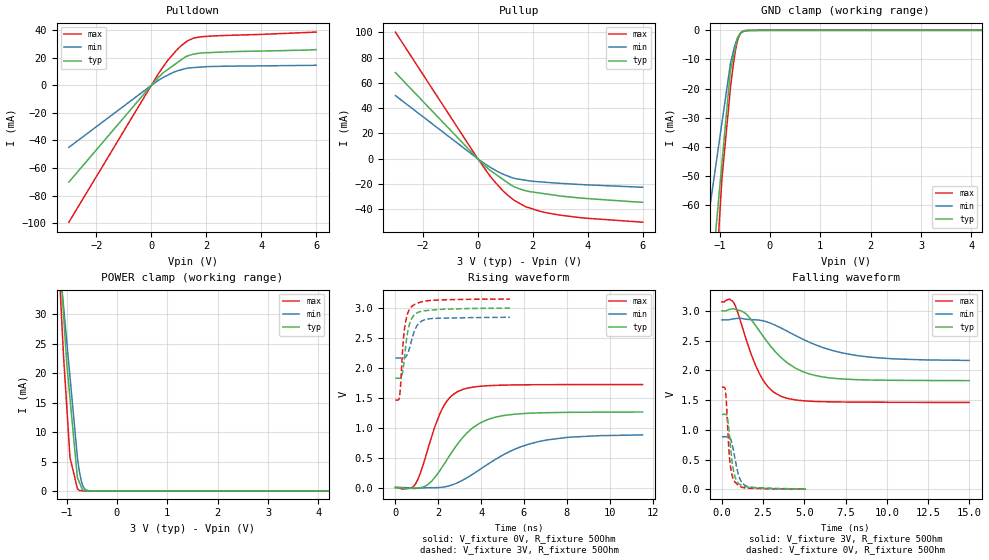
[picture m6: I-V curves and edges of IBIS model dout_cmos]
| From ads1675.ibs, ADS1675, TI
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|   dout_cmos Model
[Model]   dout_cmos
Model_type   3-state
Polarity   Non-Inverting
Vmeas = 1.5
Vref = 0
Cref = 5pF
Rref = 500
|   typ   min   max
|C_comp from frequency method(F=32MHz)
|Average
|ON state : BUFFER OUTPUT TURNED HIGH
|C_comp   7.766e-12   6.692e-12   8.884e-12
|OFF state: BUFFER IN HIGH IMPEDANCE
C_comp   5.044e-12   4.178e-12   5.758e-12
|C_comp from L-C Tank method(L=1nH)
|ON state : BUFFER OUTPUT TURNED HIGH
|Resonant Frequency(Hz)   2.79e9   3.03e9   2.58e9
|C_comp   3.257e-12   2.762e-12   3.809e-12
|OFF state: BUFFER IN HIGH IMPEDANCE
|Resonant Frequency(Hz)   2.85e9   3.13e9   2.62e9
|C_comp   3.122e-12   2.588e-12   3.694e-12
| Where nom  PVT is Nominal Process,  3V,  51C
|   Fast PVT is Strong Process,   3.15V,  -40C
|   Slow PVT is Weak Process,   2.85V,  111C
[Voltage Range]   3   2.85   3.15
|Ambient Temperature   25   85   -40
|Junction Temperature
[Temperature Range]   51   111   -40
[Pullup Reference]   3   2.85   3.15
[Pulldown Reference]   0   0   0
[Power Clamp Reference]   3   2.85   3.15
[GND Clamp Reference]   0   0   0
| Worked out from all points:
|   slope of the pulldown table from 0 to 0.45 V, typ, clamps not added: 47.8 ohm
|   slope of the pullup table from 0 to 0.45 V, typ, clamps not added: 48.9 ohm
|   GND clamp passes 1 mA (typ) near -0.59 V on its own axis
|   POWER clamp passes 1 mA (typ) near -0.72 V on its own axis
|   falling waveform, V_fixture 3V, R_fixture 50Ohm: 20-80 % time 2.31ns typ, 3.56ns min, 1.44ns max; typ from 3 V to 1.83 V
|   rising waveform, V_fixture 0V, R_fixture 50Ohm: 20-80 % time 1.64ns typ, 2.65ns min, 1.02ns max; typ from 0 V to 1.26 V
|   rising waveform, V_fixture 3V, R_fixture 50Ohm: 20-80 % time 300ps typ, 382ps min, 242ps max; typ from 1.82 V to 3 V
|   falling waveform, V_fixture 0V, R_fixture 50Ohm: 20-80 % time 326ps typ, 421ps min, 250ps max; typ from 1.26 V to 0.007 V
[Pulldown]
|   Voltage   I(typ)   I(min)   I(max)
-3V       -70.2mA    -44.95mA   -99.32mA
242.5mV   5.395mA    3.388mA    8.009mA
420mV     8.976mA    5.561mA    13.13mA
614.2mV   11.76mA    7.657mA    18.56mA
1.093V    18.63mA    11.39mA    28.92mA
1.329V    21.43mA    12.55mA    32.51mA
1.553V    22.71mA    12.94mA    34.4mA
1.906V    23.64mA    13.46mA    35.44mA
6V        25.95mA    14.6mA     38.7mA
[GND Clamp]
|   Voltage   I(typ)   I(min)   I(max)
-3V       -1.057A    -965.9mA   -1.19A
-1.385V   -127.5mA   -83.76mA   -183.3mA
-1.162V   -85.25mA   -56.89mA   -110.8mA
-954.5mV  -45.77mA   -31.82mA   -51.12mA
-786mV    -13.79mA   -11.5mA    -20.01mA
-746.6mV  -10.59mA   -8.61mA    -14.27mA
-711.9mV  -7.792mA   -6.173mA   -9.856mA
-680.4mV  -5.244mA   -4.383mA   -6.505mA
-652.1mV  -2.951mA   -3.004mA   -4.138mA
-592.2mV  -1.075mA   -1.268mA   -1.201mA
-513.4mV  -199uA     -347.9uA   -140.8uA
6V        0A         0A         0A
[Pullup]
|   Voltage   I(typ)   I(min)   I(max)
-3V       68.19mA    49.98mA    100.2mA
0V        0A         0A         0A
420mV     -8.738mA   -6.297mA   -12.9mA
554.4mV   -10.79mA   -8.014mA   -16.64mA
957.6mV   -16.93mA   -12.54mA   -26.2mA
1.317V    -22mA      -15.4mA    -32.74mA
1.764V    -25.39mA   -17.07mA   -38.09mA
2.303V    -27.26mA   -18.33mA   -41.72mA
2.974V    -29.35mA   -19.37mA   -44.5mA
3.938V    -31.41mA   -20.58mA   -47mA
6V        -34.42mA   -22.53mA   -50.15mA
[POWER Clamp]
|   Voltage   I(typ)   I(min)   I(max)
-3V       364.4mA    413.3mA    365.3mA
-1.26V    55.77mA    49.9mA     56.34mA
-1.065V   30.51mA    31.72mA    23.55mA
-996mV    21.61mA    25.32mA    14.21mA
-932.4mV  15.75mA    19.39mA    5.637mA
-786mV    2.266mA    5.745mA    431.8uA
-737.1mV  1.262mA    2.891mA    65.04uA
-701.1mV  523.4uA    1.481mA    39.31uA
-684mV    172.4uA    1.019mA    27.09uA
-661.2mV  95.5uA     587.3uA    10.79uA
-561.5mV  7.479uA    36.29uA    1.342uA
6V        0A         0A         0A
[Ramp]
R_load = 50
|   typ   min   max
dV/dt_r   0.757498/1.64022e-09   0.530712/2.66751e-09   1.0325/1.01817e-09
dV/dt_f   0.702471/2.29768e-09   0.408901/3.56008e-09   1.01274/1.44319e-09
[Falling Waveform]
V_fixture = 3V
V_fixture_min = 2.85V
V_fixture_max = 3.15V
R_fixture = 50Ohm
|   Time   V(typ)   V(min)   V(max)
0s        3V         2.85V      3.15V
440ps     3.024V     2.852V     3.199V
716ps     3.036V     2.868V     3.139V
1.368ns   2.971V     2.864V     2.613V
2.268ns   2.666V     2.845V     1.952V
2.88ns    2.434V     2.802V     1.7V
3.604ns   2.213V     2.711V     1.565V
5.408ns   1.933V     2.462V     1.482V
7.94ns    1.848V     2.262V     1.469V
15ns      1.829V     2.168V     1.462V
[Rising Waveform]
V_fixture = 0V
V_fixture_min = 0V
V_fixture_max = 0V
R_fixture = 50Ohm
|   Time   V(typ)   V(min)   V(max)
0s        2.3nV      3.017nV    1.724nV
928ps     -7.148mV   -16.41mV   53.7mV
1.5ns     46.29mV    -3.953mV   622.9mV
2.1ns     296.7mV    1.796mV    1.252V
2.5ns     518.3mV    27.13mV    1.488V
2.912ns   732.6mV    81.86mV    1.604V
3.948ns   1.078V     302.7mV    1.691V
5.032ns   1.202V     546.4mV    1.711V
7.132ns   1.251V     797.9mV    1.719V
11.54ns   1.261V     879.1mV    1.721V
[Rising Waveform]
V_fixture = 3V
V_fixture_min = 2.85V
V_fixture_max = 3.15V
R_fixture = 50Ohm
|   Time   V(typ)   V(min)   V(max)
0s        1.825V     2.164V     1.46V
200ps     1.824V     2.165V     1.537V
248ps     1.831V     2.165V     1.738V
352ps     1.962V     2.164V     2.374V
484ps     2.371V     2.183V     2.782V
620ps     2.676V     2.283V     2.951V
792ps     2.843V     2.507V     3.033V
1.044ns   2.925V     2.722V     3.082V
1.408ns   2.955V     2.807V     3.116V
5.344ns   2.997V     2.844V     3.148V
[Falling Waveform]
V_fixture = 0V
V_fixture_min = 0V
V_fixture_max = 0V
R_fixture = 50Ohm
|   Time   V(typ)   V(min)   V(max)
0s        1.262V     886.5mV    1.72V
212ps     1.264V     886.2mV    1.667V
328ps     1.207V     888mV      1.172V
420ps     1.02V      884.2mV    691.7mV
508ps     767.5mV    855.8mV    415.5mV
660ps     384.9mV    713.9mV    198.6mV
832ps     183.8mV    464.8mV    113.9mV
1.084ns   85.97mV    183.7mV    55.17mV
1.476ns   48.93mV    59.11mV    24.53mV
5.1ns     6.861mV    8.566mV    5.532mV
